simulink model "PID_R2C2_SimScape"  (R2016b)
settings: Solver=ode45  StartTime=0.0  StopTime=.25  RelTol=1e-10  EnableMultiTasking=on
libraries: fl_lib x15, nesl_utility x3

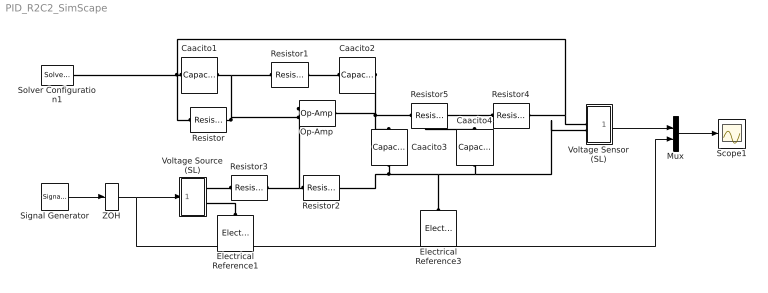
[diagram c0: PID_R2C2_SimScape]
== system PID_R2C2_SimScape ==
  Caacito1 : fl_lib/Electrical/Electrical Elements/Capacitor  c=1e-6 F  r=1e-6 Ohm  g=0 1/Ohm  i_specify=off  i_priority=None  i=0 A  v_specify=off  v_priority=None  v=0 V  vc_specify=on  vc_priority=High  vc=0 V
  Caacito2 : fl_lib/Electrical/Electrical Elements/Capacitor  c=1e-6 F  r=1e-6 Ohm  g=0 1/Ohm  i_specify=off  i_priority=None  i=0 A  v_specify=off  v_priority=None  v=0 V  vc_specify=on  vc_priority=High  vc=0 V
  Caacito3 : fl_lib/Electrical/Electrical Elements/Capacitor  c=100e-6 F  r=1e-6 Ohm  g=0 1/Ohm  i_specify=off  i_priority=None  i=0 A  v_specify=off  v_priority=None  v=0 V  vc_specify=on  vc_priority=High  vc=0 V
  Caacito4 : fl_lib/Electrical/Electrical Elements/Capacitor  c=100e-6 F  r=1e-6 Ohm  g=0 1/Ohm  i_specify=off  i_priority=None  i=0 A  v_specify=off  v_priority=None  v=0 V  vc_specify=on  vc_priority=High  vc=0 V
  Electrical Reference1 : fl_lib/Electrical/Electrical Elements/Electrical Reference
  Electrical Reference3 : fl_lib/Electrical/Electrical Elements/Electrical Reference
  Mux : Mux  Inputs=2
  Op-Amp : fl_lib/Electrical/Electrical Elements/Op-Amp  outI_specify=off  outI_priority=None  outI=0 A
  Resistor{,1..3} (4 alike) : fl_lib/Electrical/Electrical Elements/Resistor  R=1 kOhm  i_specify=off  i_priority=None  i=0 A  v_specify=off  v_priority=None  v=0 V
  Resistor4 : fl_lib/Electrical/Electrical Elements/Resistor  R=10 kOhm  i_specify=off  i_priority=None  i=0 A  v_specify=off  v_priority=None  v=0 V
  Resistor5 : fl_lib/Electrical/Electrical Elements/Resistor  R=10 kOhm  i_specify=off  i_priority=None  i=0 A  v_specify=off  v_priority=None  v=0 V
  Scope1 : Scope
  Signal Generator : SignalGenerator  WaveForm=square  Frequency=100
  Solver Configuration1 : nesl_utility/Solver Configuration  PhysicalDomain=network_engine_domain  SubClassName=solver  LeftPortType=input  RightPortType=generic  Accelerate=off  Tones=[]  Harmonics=[]  SimulateNoise=off  Profile=off  UseLocalSampling=off  EnableSwitchedLinearOptims=on  FrequencyDomain=off  UseCCode=off  RelTol=0.001  AbsTol=1e-06  MinStep=1e-09  ToWorkspace=off  RevertToSquareIcSolve=off  NumHomotopyIterations=100  PhasorMode=off  PhasorModeNumHarmonics=1  OverrideAbsTol=off  DoDC=off  ResidualTolerance=1e-4  UseLocalSolver=on  LocalSolverChoice=NE_BACKWARD_EULER_ADVANCER  LocalSolverSampleTime=.001  DoFixedCost=on  MaxNonlinIter=3  MaxModeIter=2  LinearAlgebra=Sparse  DelaysMemoryBudget=1024  AutomaticFiltering=on  FilteringTimeConstant=0.001
  Voltage Sensor (SL) : Subsystem
  Voltage Source (SL) : Subsystem
  ZOH : ZeroOrderHold  SampleTime=.001
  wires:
  Signal Generator/1 -> ZOH/1
  Mux/1 -> Scope1/1
  Voltage Sensor (SL)/1(v) -> Mux/1
  ZOH/1 -> Voltage Source (SL)/1(S), Mux/2
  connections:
  Caacito1/RConn1 -- Resistor/RConn1 -- Op-Amp/LConn2 -- Resistor1/LConn1
  Caacito1/LConn1 -- Resistor/LConn1 -- Resistor4/LConn1 -- Voltage Sensor (SL)/LConn1 -- Solver Configuration1/RConn1
  Resistor2/LConn1 -- Op-Amp/LConn1 -- Resistor3/LConn1
  Caacito2/LConn1 -- Resistor1/RConn1
  Caacito2/RConn1 -- Op-Amp/RConn1 -- Resistor5/RConn1 -- Caacito3/LConn1
  Resistor5/LConn1 -- Resistor4/RConn1 -- Caacito4/LConn1
  Caacito3/RConn1 -- Electrical Reference3/LConn1 -- Caacito4/RConn1 -- Voltage Sensor (SL)/LConn2 -- Resistor2/RConn1
  Electrical Reference1/LConn1 -- Voltage Source (SL)/RConn2
  Voltage Source (SL)/RConn1 -- Resistor3/RConn1

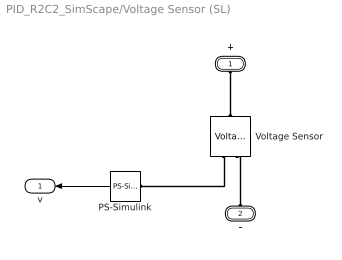
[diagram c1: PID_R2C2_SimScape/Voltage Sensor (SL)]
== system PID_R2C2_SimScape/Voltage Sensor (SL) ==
  PS-Simulink : nesl_utility/PS-Simulink Converter  PhysicalDomain=network_engine_domain  SubClassName=ps_output  LeftPortType=input  RightPortType=output  PseudoPeriodic=off  Frequencies=[]  Unit=V  AffineConversion=off
  Voltage Sensor : fl_lib/Electrical/Electrical Sensors/Voltage Sensor
  + : PMIOPort  Port=1  Side=Left
  - : PMIOPort  Port=2  Side=Left
  v : Outport
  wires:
  PS-Simulink/1 -> v/1
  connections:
  Voltage Sensor/RConn1 -- PS-Simulink/LConn1
  +/RConn1 -- Voltage Sensor/LConn1
  -/RConn1 -- Voltage Sensor/RConn2

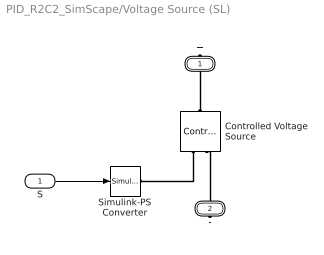
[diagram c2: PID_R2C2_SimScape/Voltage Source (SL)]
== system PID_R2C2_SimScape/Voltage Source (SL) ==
  S : Inport
  Controlled Voltage Source : fl_lib/Electrical/Electrical Sources/Controlled Voltage Source
  Simulink-PS Converter : nesl_utility/Simulink-PS Converter  PhysicalDomain=network_engine_domain  SubClassName=ps_input  LeftPortType=input  RightPortType=output  PseudoPeriodic=off  Frequencies=[]  NoiseDistribution=none  NoiseParameters=[]  Unit=V  AffineConversion=off  InputFiltering=off  SimscapeFilterOrder=1  InputFilterTimeConstant=.001  UdotUserProvided=0
  + : PMIOPort  Port=1  Side=Right
  - : PMIOPort  Port=2  Side=Right
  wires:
  S/1 -> Simulink-PS Converter/1
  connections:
  Controlled Voltage Source/RConn1 -- Simulink-PS Converter/RConn1
  -/RConn1 -- Controlled Voltage Source/RConn2
  +/RConn1 -- Controlled Voltage Source/LConn1
